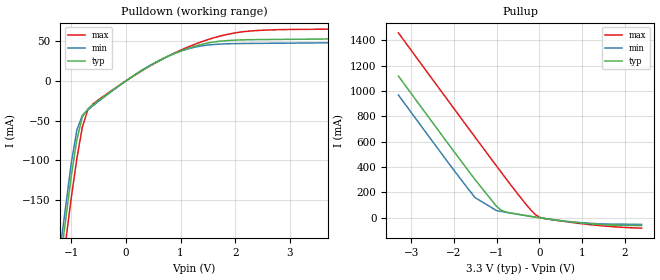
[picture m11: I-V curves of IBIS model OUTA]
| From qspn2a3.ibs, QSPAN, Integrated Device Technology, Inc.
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|   Model OUTA
[Model]   OUTA
Model_type   Output
Polarity   Non-Inverting
C_comp   5.00pF   5.00pF   5.00pF
[Voltage Range]   3.3000V   3.0000V   4.0000V
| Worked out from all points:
|   slope of the pulldown table from 0 to 0.495 V, typ, clamps not added: 23.4 ohm
|   slope of the pullup table from 0 to 0.495 V, typ, clamps not added: 21.1 ohm
[Pulldown]
| voltage   I(typ)   I(min)   I(max)
-3.3V     -1.412A    -1.395A    -1.438A
-1.5V     -386.4mA   -368.6mA   -415.1mA
-1V       -118.7mA   -102.4mA   -146.1mA
-900mV    -74.09mA   -62.07mA   -98.14mA
-800mV    -45.29mA   -43.39mA   -58.29mA
-700mV    -35.4mA    -36.6mA    -36.58mA
-600mV    -29.77mA   -31.03mA   -28.79mA
100mV     4.634mA    4.818mA    4.49mA
600mV     25mA       25.47mA    24.92mA
1.2V      42.38mA    41.45mA    44.46mA
1.9V      50.9mA     46.76mA    59.14mA
3.7V      52.82mA    47.89mA    65.08mA
[Pullup]
| voltage   I(typ)   I(min)   I(max)
-3.3V     1.118A     968.3mA    1.459A
-2.1V     568.9mA    420.5mA    908.2mA
-1.5V     298.7mA    157.7mA    634.1mA
-1V       89.65mA    55.78mA    407.7mA
-900mV    60.99mA    49.9mA     362.8mA
-400mV    21.53mA    21.32mA    143.3mA
-100mV    5.24mA     5.171mA    27.56mA
0V        793.5pA    1.407nA    4.425mA
100mV     -5.099mA   -5.005mA   -4.766mA
700mV     -31.76mA   -30.3mA    -34.8mA
1.5V      -55.13mA   -49.3mA    -64.86mA
2.4V      -61.9mA    -52.42mA   -82.69mA
[Ramp]
| variable   typ   min   max
dV/dt_r   1.3368/0.4974n   1.1952/0.4909n   1.6692/0.4326n
dV/dt_f   1.2654/0.2783n   1.1628/0.2569n   1.5090/0.3582n
R_load = 50.0000
| End [Model] OUTA
